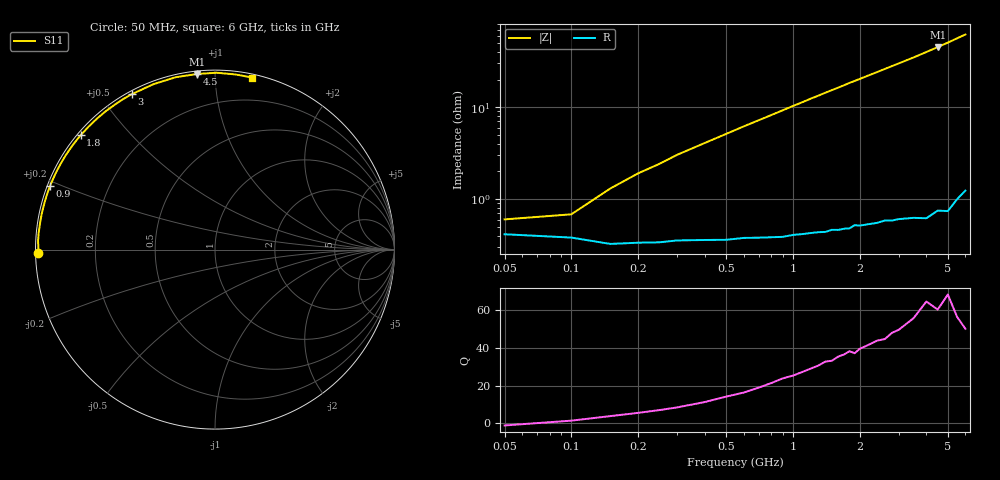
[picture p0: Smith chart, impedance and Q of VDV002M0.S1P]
! Infineon Technologies  Discrete & RF Semiconductors
! BBY 55-03
! Si Tuning Diode in SOD323
! VR =
! S-Parameters:  June  1999
# GHz  S  MA  R  50
!  f  S11
! GHz  MAG  ANG
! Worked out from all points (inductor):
!   34 points, 50 MHz to 6 GHz, reference 50 ohm
!   read as one part to ground: L = 1.49 nH near 150 MHz
!   highest Q = 64.4 at 4.5 GHz (marker M1), where L = 1.6 nH
!   S11 on the Smith chart (normalised r, x): 50 MHz: 0.01, -0.01; 900 MHz: 0.01, +0.19; 1.8 GHz: 0.01, +0.37; 3 GHz: 0.01, +0.60; 4.5 GHz: 0.02, +0.90; 6 GHz: 0.02, +1.24
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0.05  0.9835 -179.0
0.1  0.9849 178.7
0.15  0.9871 177.1
0.2  0.9867 175.7
0.25  0.9866 174.5
0.3  0.9859 173.1
0.5  0.9858 168.3
0.6  0.9852 165.9
0.8  0.9851 161.3
0.9  0.9851 159.0
1  0.9845 156.7
1.1  0.9843 154.5
1.2  0.984 152.2
1.4  0.9839 147.9
1.6  0.9834 143.8
1.8  0.9832 139.6
2  0.9825 135.8
2.2  0.9823 132.0
2.4  0.9823 128.4
2.6  0.9818 124.8
2.8  0.9823 121.4
3  0.9823 118.1
3.5  0.9833 110.3
4  0.985 102.8
4.5  0.9836 95.8
5  0.9854 89.4
5.5  0.9825 83.3
6  0.9807 77.8
